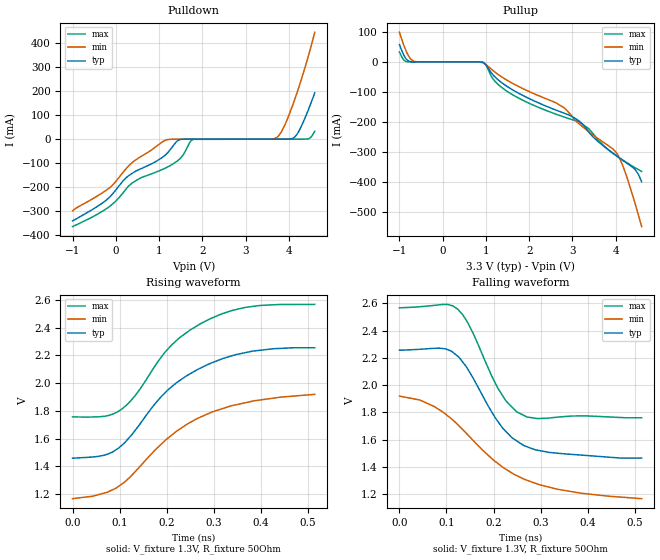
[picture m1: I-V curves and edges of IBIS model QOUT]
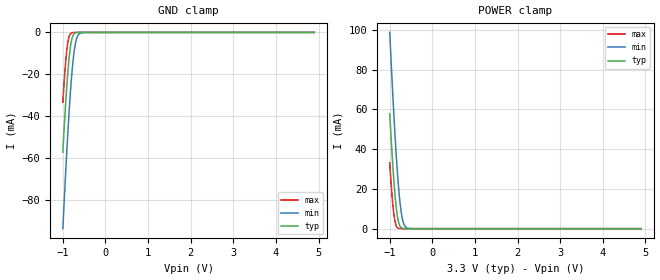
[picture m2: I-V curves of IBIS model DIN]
|Texas Instruments Incorporated
|LVTTL/LVCOMS to differential LVPECL Buffer
| Marketing part#   Voltage Range   Package-type   #pins
| SN65EPT22DGKR   3.0 to 3.6V   MSOP   8
| SN65EPT22DR   3.0 to 3.6V   SOIC   8
[IBIS Ver]   3.2
[File name]   sn65ept22.ibs
[File Rev]   1.0
[Date]   11/04/2010
[Source]   Texas Instruments Incorporated.
|   Analog-eLab, HPA
|   12500 TI Blvd
|   Dallas, TX -75243
|   For Support e-mail: elab_ibis@list.ti.com
[Notes]
|-Revision History:
| 1.0: 11/04/2010
| - Initial version of the model
| - Initial Model generated from simulations in TISPICE
| - No syntax warnings or errors based on the committee parser checker
[Disclaimer]
 This product is designed as an aid for customers of Texas Instruments.
 No warranties, either expressed or implied, with respect to this third
 party software (if any) or with respect to its fitness for any
 particular purpose is claimed by Texas Instruments or the author. The
 software (if any) is provided solely on an "as is" basis. The entire
 risk as to its quality and performance is with the customer
[Copyright] (C) Copyright 2010 Texas Instruments Incorporated.
   All rights reserved.
|   Component   SN65EPT22DGKR
[Component]   SN65EPT22DGKR
[Manufacturer]   Texas Instruments Incorporated
[Package]
|   typ   min   max
R_pkg   0.2341   0.1409   0.2717
L_pkg   0.842nH   0.72420nH   0.90698nH
C_pkg   0.405pF   0.3879pF   0.43798pF
[Pin] signal_name   model_name   R_pin   L_pin   C_pin
1   Q0   QOUT   0.27170  0.90498nH  0.38798pF
2   Q0B   QOUT   0.25240  0.84957nH  0.40564pF
3   Q1   QOUT   0.25240  0.84985nH  0.40565pF
4   Q1B   QOUT   0.27170  0.90697nH  0.38809pF
5   GND   GND   0.27170  0.90698nH  0.38874pF
6   D1   DIN   0.14095  0.72489nH  0.43798pF
7   D0   DIN   0.14095  0.72420nH  0.43795pF
8   VCC   POWER   0.27170  0.90497nH  0.38864pF
|   Component   SN65EPT22DR
[Component]   SN65EPT22DR
[Manufacturer]   Texas Instruments Incorporated
[Package]
|   typ   min   max
R_pkg   0.14515   0.0914   0.17317
L_pkg   1.186nH   0.9612nH   1.287nH
C_pkg   0.4386pF   0.3992pF   0.46414pF
[Pin] signal_name   model_name   R_pin   L_pin   C_pin
1   Q0   QOUT   0.15806  1.28353nH  0.46339pF
2   Q0B   QOUT   0.17315  1.21037nH  0.38922pF
3   Q1   QOUT   0.17317  1.21250nH  0.38980pF
4   Q1B   QOUT   0.15802  1.28448nH  0.46211pF
5   GND   GND   0.15806  1.28701nH  0.46414pF
6   D1   DIN   0.09143  0.96935nH  0.43901pF
7   D0   DIN   0.09140  0.96121nH  0.43785pF
8   VCC   POWER   0.15806  1.28355nH  0.46396pF
[Diff Pin]  inv_pin  vdiff  tdelay_typ tdelay_min tdelay_max
1   2   NA   0   0   0
3   4   NA   0   0   0
| Models and submodels in the file (2): QOUT (Output), DIN (Input)
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|   Model   QOUT
[Model]   QOUT
Model_type   Output
Polarity   Non-Inverting
Enable   Active-High
Vmeas = 1.85
Vref = 1.3
Cref = 1pF
Rref = 50
|   typ   min   max
C_comp   0.53258pF   0.48373pF   0.61904pF
[Voltage Range]   3.3   3   3.6
[Temperature Range]   27   125   -40
[Pullup Reference]   3.3   3   3.6
[Pulldown Reference]   0   0   0
[Power Clamp Reference]   3.3   3   3.6
[GND Clamp Reference]   0   0   0
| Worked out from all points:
|   slope of the pulldown table from 0 to 0.495 V, typ, clamps not added: 6.06 ohm
|   falling waveform, V_fixture 1.3V, R_fixture 50Ohm: 20-80 % time 88.1ps typ, 156ps min, 66.6ps max; typ from 2.26 V to 1.46 V
|   rising waveform, V_fixture 1.3V, R_fixture 50Ohm: 20-80 % time 141ps typ, 160ps min, 126ps max; typ from 1.46 V to 2.25 V
[Pulldown]
|   Voltage   I(typ)   I(min)   I(max)
-1V       -341mA     -299.1mA   -364.7mA
-129.8mV  -239.3mA   -200.8mA   -278.6mA
164.9mV   -174.5mA   -138.9mA   -224.9mA
417.5mV   -138.1mA   -92.18mA   -178.4mA
1.063V    -77.74mA   -13.12mA   -127.5mA
1.47V     -2.211mA   -914.6nA   -83.61mA
1.793V    -14.02nA   -95.51pA   -744.5uA
3.73V     5.26nA     8.138mA    13.18pA
3.912V    5.945uA    60.92mA    15.65pA
4.179V    17.58mA    187.9mA    3.515nA
4.46V     126.4mA    351.9mA    2.101mA
4.6V      193.4mA    446mA      33.07mA
[GND Clamp]
|   Voltage   I(typ)   I(min)   I(max)
-1V       0A         0A         0A
3.3V      0A         0A         0A
4.6V      0A         0A         0A
[Pullup]
|   Voltage   I(typ)   I(min)   I(max)
-1V       57.8mA     98.7mA     33.07mA
-845.6mV  10.22mA    36.4mA     1.283mA
-663.2mV  41.66uA    2.041mA    229nA
936.8mV   -2.358mA   -3.521mA   -1.025mA
1.189V    -47.24mA   -31.73mA   -61.27mA
1.47V     -79.77mA   -59.44mA   -96.13mA
2.804V    -170.4mA   -152.4mA   -183.2mA
3.154V    -196.9mA   -206.1mA   -201.4mA
3.379V    -233.7mA   -232.7mA   -222.7mA
4.039V    -315mA     -307.3mA   -314.5mA
4.432V    -355.5mA   -463.3mA   -350.8mA
4.6V      -399.3mA   -548.3mA   -364.6mA
[POWER Clamp]
|   Voltage   I(typ)   I(min)   I(max)
-1V       0A         0A         0A
3.3V      0A         0A         0A
4.6V      0A         0A         0A
[Ramp]
R_load = 50
|   typ   min   max
dV/dt_r   0.478158/1.40858e-010  0.451792/1.60349e-010  0.487339/1.25669e-010
dV/dt_f   0.47491/8.80713e-011  0.451792/1.55827e-010  0.484334/6.66111e-011
[Falling Waveform]
V_fixture = 1.3V
V_fixture_min = 1V
V_fixture_max = 1.6V
R_fixture = 50Ohm
C_fixture = 0F
|   Time   V(typ)   V(min)   V(max)
0s        2.256V     1.919V     2.567V
73.72ps   2.269V     1.843V     2.584V
97.96ps   2.265V     1.787V     2.591V
124.2ps   2.211V     1.709V     2.556V
145.3ps   2.116V     1.634V     2.457V
196.2ps   1.803V     1.461V     2.066V
226.4ps   1.659V     1.381V     1.883V
271.2ps   1.547V     1.301V     1.765V
385.7ps   1.486V     1.206V     1.773V
514.8ps   1.464V     1.166V     1.759V
[Rising Waveform]
V_fixture = 1.3V
V_fixture_min = 1V
V_fixture_max = 1.6V
R_fixture = 50Ohm
C_fixture = 0F
|   Time   V(typ)   V(min)   V(max)
0s        1.458V     1.166V     1.756V
66.1ps    1.479V     1.205V     1.76V
103.1ps   1.547V     1.267V     1.809V
134.7ps   1.666V     1.367V     1.917V
173ps     1.841V     1.508V     2.112V
208.9ps   1.969V     1.62V      2.27V
248.8ps   2.065V     1.714V     2.381V
293.6ps   2.143V     1.787V     2.466V
365.8ps   2.219V     1.857V     2.546V
514.8ps   2.255V     1.919V     2.568V
|   Model   DIN
[Model]   DIN
Model_type   Input
Vinl = 0.8
Vinh = 2
|   typ   min   max
C_comp   0.38647pF   0.33500pF   0.45077pF
[Voltage Range]   3.3   3   3.6
[Temperature Range]   27   125   -40
[Power Clamp Reference]   3.3   3   3.6
[GND Clamp Reference]   0   0   0
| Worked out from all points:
|   GND clamp passes 1 mA (typ) near -0.75 V on its own axis
|   POWER clamp passes 1 mA (typ) near -0.75 V on its own axis
[GND Clamp]
|   Voltage   I(typ)   I(min)   I(max)
-1V       -57.1mA    -93.59mA   -33.21mA
-940.7mV  -35.9mA    -69.49mA   -15.5mA
-911.1mV  -26.54mA   -58.16mA   -8.938mA
-881.4mV  -18.35mA   -47.44mA   -4.409mA
-851.8mV  -11.62mA   -37.48mA   -1.847mA
-822.1mV  -6.595mA   -28.43mA   -684.4uA
-792.5mV  -3.32mA    -20.5mA    -245.4uA
-762.8mV  -1.493mA   -13.88mA   -89.29uA
-733.2mV  -616uA     -8.733mA   -31.58uA
-673.9mV  -92.18uA   -2.736mA   -6.735uA
-614.6mV  -19.06uA   -673.4uA   -4.887uA
4.9V      0A         0A         0A
[POWER Clamp]
|   Voltage   I(typ)   I(min)   I(max)
-1V       57.8mA     98.7mA     33.07mA
-940.7mV  36.06mA    72.59mA    15.2mA
-911.1mV  26.52mA    60.43mA    8.622mA
-881.4mV  18.21mA    49.01mA    4.113mA
-851.8mV  11.42mA    38.46mA    1.601mA
-822.1mV  6.387mA    28.96mA    505.9uA
-792.5mV  3.137mA    20.7mA     133.9uA
-762.8mV  1.354mA    13.88mA    32.09uA
-703.5mV  185.9uA    4.944mA    1.704uA
-673.9mV  62.37uA    2.615mA    390.1nA
-614.6mV  6.493uA    605uA      20.48nA
4.9V      0A         0A         0A
